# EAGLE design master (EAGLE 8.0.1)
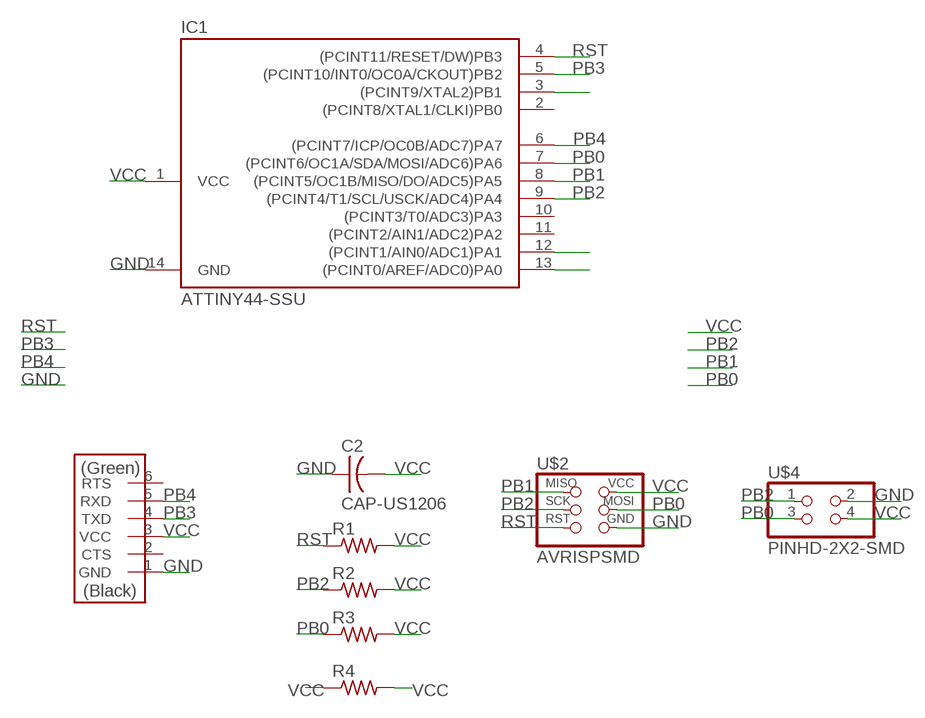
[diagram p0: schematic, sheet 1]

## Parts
C2  CAP-US1206  [C1206]
IC1  ATTINY44-SSU  [SOIC14]
R1  RES-US1206  [R1206]
R2  RES-US1206  [R1206]
R3  RES-US1206  [R1206]
R4  RES-US1206  [R1206]
U$2  AVRISPSMD  [2X03SMD]
U$3  FTDI-SMD-HEADER  [1X06SMD]
U$4  PINHD-2X2-SMD  [2X02SMD]

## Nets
GND: C2.1 IC1.14(GND) U$2.6(GND) U$3.1(GND) U$4.2
N$5: IC1.3((PCINT9/XTAL2)PB1)
N$13: IC1.12((PCINT1/AIN0/ADC1)PA1)
N$14: IC1.13((PCINT0/AREF/ADC0)PA0)
PB0: IC1.7((PCINT6/OC1A/SDA/MOSI/ADC6)PA6) R3.1 U$2.4(MOSI) U$4.3
PB1: IC1.8((PCINT5/OC1B/MISO/DO/ADC5)PA5) U$2.1(MISO)
PB2: IC1.9((PCINT4/T1/SCL/USCK/ADC4)PA4) R2.1 U$2.3(SCK) U$4.1
PB3: IC1.5((PCINT10/INT0/OC0A/CKOUT)PB2) U$3.4(TXD)
PB4: IC1.6((PCINT7/ICP/OC0B/ADC7)PA7) U$3.5(RXD)
RST: IC1.4((PCINT11/RESET/DW)PB3) R1.1 U$2.5(RST)
VCC: C2.2 IC1.1(VCC) R1.2 R2.2 R3.2 R4.1 R4.2 U$2.2(VCC) U$3.3(VCC) U$4.4
Unconnected: IC1.2((PCINT8/XTAL1/CLKI)PB0) IC1.10((PCINT3/T0/ADC3)PA3) IC1.11((PCINT2/AIN1/ADC2)PA2) U$3.2(CTS) U$3.6(RTS)

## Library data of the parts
C2 = fab:CAP-US
IC1 = fab:ATTINY44
R1-R4 = fab:RES-US: Resistor (US Symbol)
U$2 = fab:AVRISP
U$3 = fab:FTDI-SMD-HEADER
U$4 = fab:PINHD-2X2-SMD

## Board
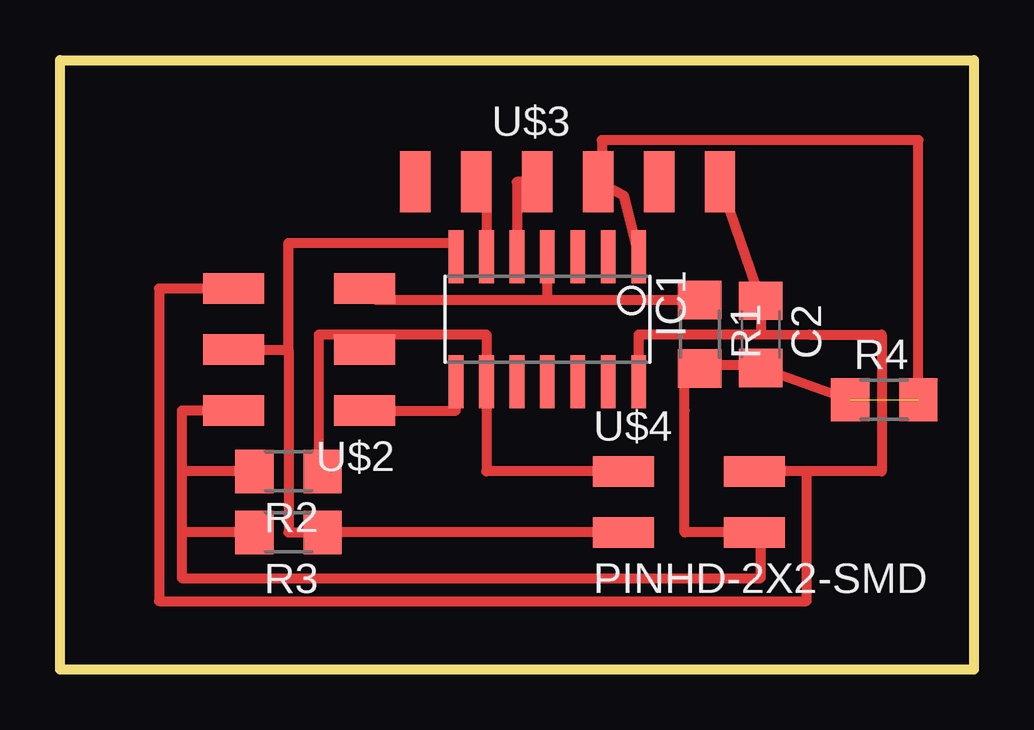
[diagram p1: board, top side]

Size 38.1 x 25.4 mm. Coordinates in mm from the lower left corner, seen from the top.
Outline: 38.1,0 0,0 0,25.4 38.1,25.4 38.1,0
Copper layers (1*16): Top 0.035mm / dielectric 1.5mm / Bottom 0.035mm
Design rules "default": minimum track width 10mil, minimum drill 24mil, track to track 8mil, track to pad 8mil, pad to pad 8mil, via to via 8mil, smd to smd 8mil, copper to edge 40mil, drill to drill 8mil, minimum pad ring 10mil, minimum via ring 8mil, stop-mask expansion 4mil, vias tented up to drill 0mil, thermal gap 10mil

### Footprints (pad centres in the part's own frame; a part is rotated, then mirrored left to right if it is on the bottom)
C1206 = smd 1.6 x 1.8: 1 -1.4,0; 2 1.4,0
SOIC14 = smd 0.61 x 2.21: 1 -3.81,-2.603; 2 -2.54,-2.603; 3 -1.27,-2.603; 4 0,-2.603; 5 1.27,-2.603; 6 2.54,-2.603; 7 3.81,-2.603; 8 3.81,2.603; 9 2.54,2.603; 10 1.27,2.603; 11 0,2.603; 12 -1.27,2.603; 13 -2.54,2.603; 14 -3.81,2.603
R1206 = smd 1.6 x 1.803: 1 -1.422,0; 2 1.422,0
2X03SMD = smd 2.54 x 1.27: 1 -2.54,2.54; 2 2.92,2.54; 3 -2.54,0; 4 2.92,0; 5 -2.54,-2.54; 6 2.92,-2.54
1X06SMD = smd 2.54 x 1.27: 1 0,6.35; 2 0,3.81; 3 0,1.27; 4 0,-1.27; 5 0,-3.81; 6 0,-6.35
2X02SMD = smd 2.54 x 1.27: 1 -2.54,1.27; 2 2.92,1.27; 3 -2.54,-1.27; 4 2.92,-1.27

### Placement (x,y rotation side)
C2  29.21,13.97 270 top
IC1  20.32,14.61 180 top
R1  26.67,13.97 270 top
R2  9.53,8.25 180 top
R3  9.53,5.71 180 top
R4  34.36,11.24 0 top
U$2  10.16,13.33 180 top
U$3  21.16,20.32 270 top
U$4  26.04,6.99 0 top

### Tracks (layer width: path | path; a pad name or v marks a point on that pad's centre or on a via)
GND
  Top 0.406: U$2.6 4.13,15.87 4.13,2.86 31.11,2.86 31.11,8.25 | 31.11,8.25 U$4.2 | IC1.14 24.13,13.97 29.21,13.97 | 29.21,13.97 C2.1 U$3.1 | 29.21,13.97 31.24,13.96 34.26,13.96 34.26,8.26 31.11,8.26 31.11,8.25
PB0
  Top 0.406: U$4.3 R3.1 9.53,5.71 9.53,13.33 | U$2.4 9.53,13.33 | 9.53,13.33 9.53,17.78 16.51,17.78 IC1.7
PB1
  Top 0.406: IC1.8 16.51,10.79 U$2.1
PB2
  Top 0.406: R2.1 10.79,8.25 10.79,13.97 12.7,13.97 | U$2.3 12.7,13.97 | U$4.1 17.78,8.25 IC1.9 17.78,13.97 12.7,13.97
PB3
  Top 0.406: U$3.4 19.05,20.32 IC1.5
PB4
  Top 0.406: U$3.5 17.78,20.32 IC1.6
RST
  Top 0.406: R1.1 20.32,15.39 | 20.32,15.39 13.18,15.39 U$2.5 | 20.32,15.39 IC1.4
VCC  (1 unrouted)
  Top 0.406: U$2.2 5.08,10.79 5.08,8.25 | 5.08,8.25 5.08,5.71 | 5.08,5.71 5.08,3.81 29.21,3.81 29.21,5.46 U$4.4 26.04,5.71 26.04,10.79 | R2.2 5.08,8.25 | R3.2 5.08,5.71 | 26.04,10.79 26.04,12.7 27.3,12.7 | 26.01,10.82 26.04,10.79 | 27.3,12.7 29.71,12.7 C2.2 R4.1 | R1.2 27.3,12.7 | IC1.1 23.49,19.76 U$3.3 22.59,20.32 22.59,22.06 35.78,22.06 R4.2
